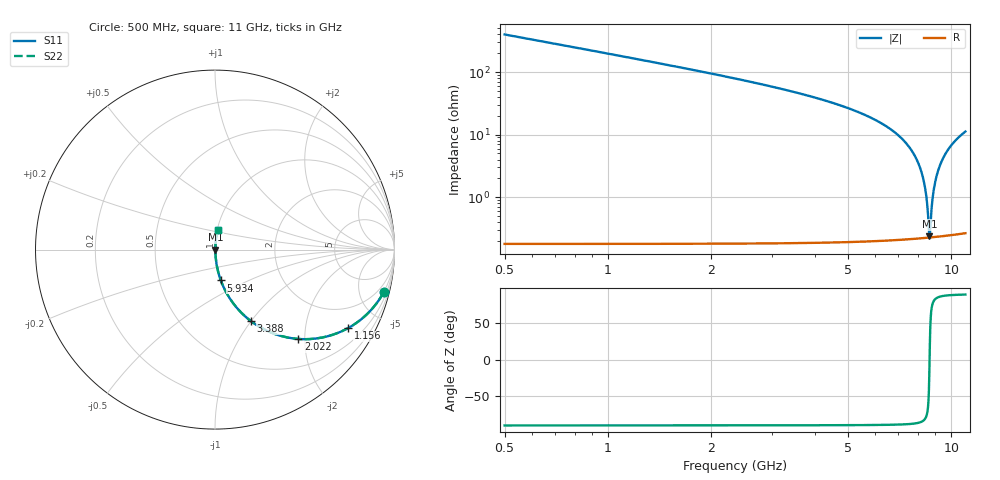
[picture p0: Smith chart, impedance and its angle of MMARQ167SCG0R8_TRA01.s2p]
! MMARQ167SCG0R8_TRA01  S-PARAMETER MODEL  ( General Type )
! Model Generated by TAIYO YUDEN Corporation (http://www.ty-top.com)
! Version 1.0
! TAIYO YUDEN Control No. 150609
! Copyright(c) 2015 TAIYO YUDEN CO.,LTD. All Rights Reserved.
! Product Description (link to TY-COMPAS)
! https://ds.yuden.co.jp/TYCOMPAS/or/detail?pn=MMARQ167SCG0R8BTRA01&u=M
! Products Name : Multilayer Ceramic Capacitors
! Characteristics :
!  Capacitance : 0.8 pF , Rated Voltage : 250V , TCC : CG / C0G
!  Case Size : 1.6 x 0.8 / 0.063 x 0.031 [mm/inch] , Thickness : 0.7 / 0.028 [mm/inch]
!  (Conditions: Temperature = 25 degC , DC Bias Current/Voltage = 0A / 0V)
! External Node Assignments :
!  1  o---| |---o  2
! GND o---------o GND
! Frequency Range : 500MHz  -  11GHz  [ 401 STEP ]
# MHz S RI R 50
! Freq[MHz].  S11 Real  S11 Imag  S21 Real  S21 Imag  S12 Real  S12 Imag  S22 Real  S22 Imag
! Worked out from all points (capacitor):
!   401 points, 500 MHz to 11 GHz, reference 50 ohm
!   read as one part in series: C = 798 fF near 552.5 MHz
!   lowest |Z| = 237 mohm at 8.637 GHz (marker M1)
!   series resonance near 8.651 GHz, so ESL is about 420 pH
!   S11 on the Smith chart (normalised r, x): 500 MHz: 1.00, -7.95; 1.156 GHz: 1.00, -3.39; 2.022 GHz: 1.00, -1.86; 3.388 GHz: 1.00, -1.00; 5.934 GHz: 1.00, -0.36; 11 GHz: 1.01, +0.22
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500  0.9404 -0.2365  0.0596 0.2365  0.0596 0.2365  0.9404 -0.2365
815  0.8545 -0.3522  0.1455 0.3522  0.1455 0.3522  0.8545 -0.3522
1156.25  0.7414 -0.4373  0.2586 0.4373  0.2586 0.4373  0.7414 -0.4373
2022.5  0.4651 -0.4978  0.5349 0.4978  0.5349 0.4978  0.4651 -0.4978
2258.75  0.404 -0.4896  0.596 0.4896  0.596 0.4896  0.404 -0.4896
3387.5  0.2 -0.3981  0.8 0.3981  0.8 0.3981  0.2 -0.3981
4017.5  0.1329 -0.3371  0.8671 0.3371  0.8671 0.3371  0.1329 -0.3371
5750  0.0379 -0.186  0.9621 0.186  0.9621 0.186  0.0379 -0.186
5933.75  0.0325 -0.1719  0.9675 0.1719  0.9675 0.1719  0.0325 -0.1719
6826.25  0.014 -0.1085  0.986 0.1085  0.986 0.1085  0.014 -0.1085
7508.75  0.00637 -0.065  0.9936 0.065  0.9936 0.065  0.00637 -0.065
7955  0.00366 -0.0385  0.9963 0.0385  0.9963 0.0385  0.00366 -0.0385
8270  0.00264 -0.0207  0.9974 0.0207  0.9974 0.0207  0.00264 -0.0207
8453.75  0.00235 -0.0106  0.9976 0.0106  0.9976 0.0106  0.00235 -0.0106
8637.5  0.00226 -0.000698  0.9977 0.000698  0.9977 0.000698  0.00226 -0.000698
8690  0.00228 0.00209  0.9977 -0.00209  0.9977 -0.00209  0.00228 0.00209
8795  0.00234 0.0076  0.9977 -0.0076  0.9977 -0.0076  0.00234 0.0076
8900  0.00247 0.0131  0.9975 -0.0131  0.9975 -0.0131  0.00247 0.0131
9057.5  0.00277 0.0211  0.9972 -0.0211  0.9972 -0.0211  0.00277 0.0211
9267.5  0.00336 0.0316  0.9966 -0.0316  0.9966 -0.0316  0.00336 0.0316
9950  0.00661 0.0642  0.9934 -0.0642  0.9934 -0.0642  0.00661 0.0642
11000  0.0149 0.11  0.9851 -0.11  0.9851 -0.11  0.0149 0.11
